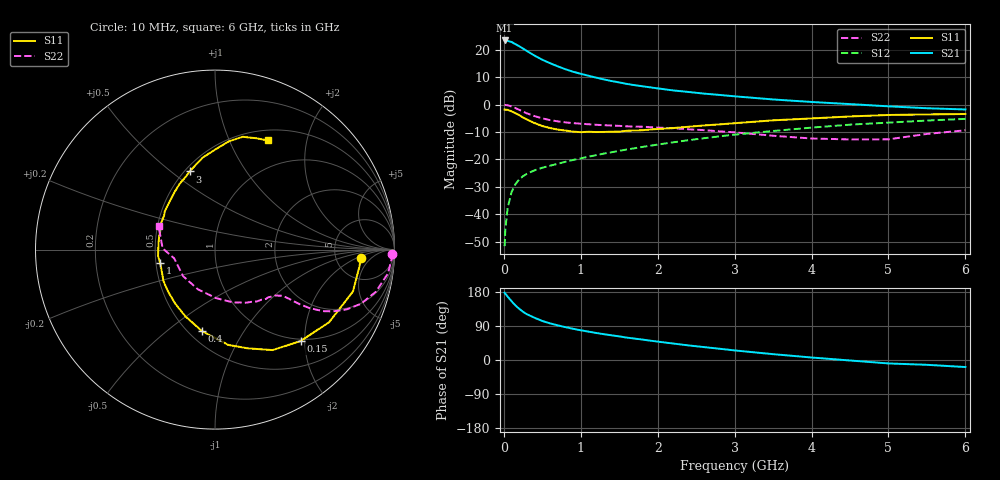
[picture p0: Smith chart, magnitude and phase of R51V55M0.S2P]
! SIEMENS Small Signal Semiconductors
! BFR183
! Si NPN RF Bipolar Junction Transistor in SOT23
! VCE = 1.5 V  IC = 5 mA
! Common Emitter S-Parameters:  May  1996
# GHz  S  MA  R  50
!  f  S11  S21  S12  S22
! GHz  MAG  ANG  MAG  ANG  MAG  ANG  MAG  ANG
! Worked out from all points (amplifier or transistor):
!   36 points, 10 MHz to 6 GHz, reference 50 ohm
!   highest |S21| = 23.4 dB at 10 MHz (marker M1)
!   |S21| within 3 dB of that: start of sweep to 251.7 MHz
!   unconditionally stable (mu >= 1): 979.2 MHz to 2.717 GHz
!   at 250 MHz: K = 0.43, MSG = 23.3 dB, |S12| = -26.1 dB
!   at 1.4 GHz: K = 1.07, MAG = 11.4 dB, |S12| = -17.4 dB
!   at 6 GHz: K = 0.91, MSG = 1.7 dB, |S12| = -5.2 dB
!   S11 on the Smith chart (normalised r, x): 10 MHz: 9.01, -2.58; 150 MHz: 0.96, -1.91; 400 MHz: 0.58, -0.67; 1 GHz: 0.53, -0.09; 3 GHz: 0.53, +0.58; 6 GHz: 0.63, +1.40
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0.01  0.814 -3.4  14.86 177.7  0.0026 87.6  0.9889 -1.5
0.02  0.8102 -6.7  14.72 174.7  0.0054 81.8  0.9848 -3.2
0.05  0.8033 -16.9  14.58 167.2  0.0131 81.4  0.973 -7.8
0.1  0.7536 -32.5  13.96 155.2  0.0252 73.7  0.9265 -14.7
0.15  0.6978 -46.9  12.73 144.1  0.0352 67.9  0.8658 -20.5
0.2  0.6452 -60.2  11.66 135.1  0.0432 63.1  0.8043 -24.5
0.25  0.5793 -71.7  10.56 127.1  0.0494 59.1  0.7426 -27.6
0.3  0.5361 -82.1  9.511 120.8  0.0546 57.5  0.6923 -29.7
0.4  0.4602 -99.0  7.857 111.4  0.0632 55.2  0.6167 -31.8
0.5  0.4067 -114.0  6.603 103.0  0.0704 53.9  0.5614 -32.8
0.6  0.3741 -126.3  5.717 96.7  0.0766 53.9  0.5219 -33.3
0.8  0.3368 -148.4  4.435 86.7  0.0903 54.8  0.4743 -34.0
1  0.3143 -166.0  3.653 78.4  0.1043 56.1  0.4487 -34.9
1.1  0.3193 -173.7  3.367 74.9  0.1119 56.6  0.438 -35.9
1.3  0.3171 172.7  2.889 68.2  0.1276 57.2  0.4211 -37.5
1.6  0.3335 156.2  2.389 59.1  0.1517 57.2  0.4017 -41.2
2.2  0.3731 131.4  1.818 43.5  0.2049 55.0  0.371 -51.1
3  0.4578 108.0  1.419 25.3  0.2832 48.3  0.3119 -70.9
3.5  0.5168 97.7  1.244 15.4  0.3304 42.7  0.2702 -88.9
4.5  0.6083 82.7  1.023 -1.3  0.4308 30.4  0.2314 -140.4
5.5  0.6621 69.5  0.86 -12.7  0.5123 17.9  0.2918 178.7
6  0.6747 64.3  0.816 -18.6  0.5492 9.8  0.3401 157.5
